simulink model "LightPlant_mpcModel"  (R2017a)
settings: Solver=VariableStepAuto  StartTime=0.0  StopTime=100  RelTol=1e-3
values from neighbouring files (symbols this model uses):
  baud = 250000    [init.m]    (also in steadyState.m; MISOcontrol.m; MISO_demo.m; runSteptest.m)
  com = 'COM4'    [init.m]    (also in steadyState.m; MISOcontrol.m; MISO_demo.m; runSteptest.m)
  fixed_u1 = 0    [init.m]    (also in MISOcontrol.m; MISO_demo.m; SISOcontrol.m)
  fixed_u2 = 0    [init.m]    (also in MISOcontrol.m; MISO_demo.m; SISOcontrol.m)
  fixed_u3 = 0    [init.m]    (also in MISOcontrol.m; MISO_demo.m; SISOcontrol.m)
  fTf = 0.1    [init.m]    (also in steadyState.m; MISOcontrol.m; MISO_demo.m; runSteptest.m)
  fTl = 0.05    [init.m]    (also in steadyState.m; MISOcontrol.m; MISO_demo.m; runSteptest.m)
  fTt = 0.05    [init.m]    (also in steadyState.m; MISOcontrol.m; MISO_demo.m; runSteptest.m)
  step_ys1_1 = +0    (= 0)    [init.m]    (also in LightPlantMPC.m = 1; MIMOcontrol.m = -2)
  step_ys1_2 = -0    (= 0)    [init.m]    (also in LightPlantMPC.m = -1; MIMOcontrol.m)
  step_ys2_1 = 0    [init.m]    (also in LightPlantMPC.m = 5; MIMOcontrol.m = -20)
  step_ys2_2 = 0    [init.m]    (also in LightPlantMPC.m = -5; MIMOcontrol.m = 10)
  stepTime_ys1_1 = 0    [init.m]    (also in LightPlantMPC.m = 30; MIMOcontrol.m = 60)
  stepTime_ys1_2 = 0    [init.m]    (also in LightPlantMPC.m = 70; MIMOcontrol.m)
  stepTime_ys2_1 = 0    [init.m]    (also in LightPlantMPC.m = 20; MIMOcontrol.m = 30)
  stepTime_ys2_2 = 0    [init.m]    (also in LightPlantMPC.m = 50; MIMOcontrol.m = 90)
  Ts = 0.1    [init.m]    (also in steadyState.m; identification.m; MISOcontrol.m; MISO_demo.m)
undefined symbols (not defined in the file or in its folder): A, B, C, D, stst
libraries: mpclib x1, tom_lib x1

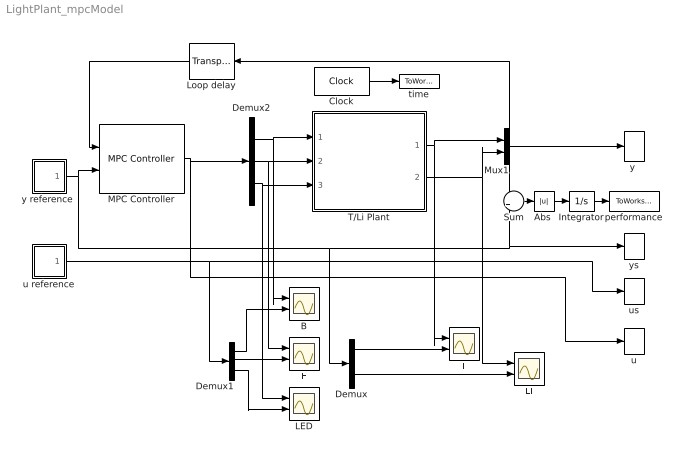
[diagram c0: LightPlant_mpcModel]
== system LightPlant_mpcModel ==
  "Abs " : Abs  ZeroCross=off
  B : Scope  NumInputPorts=2
  Clock : Clock
  Demux : Demux  Outputs=2
  Demux1 : Demux  Outputs=3
  Demux2 : Demux  Outputs=3
  F : Scope  NumInputPorts=2
  Integrator : Integrator  ZeroCross=off
  LED : Scope  NumInputPorts=2
  LI : Scope  NumInputPorts=2
  Loop delay : TransportDelay  DelayTime=0.1
  MPC Controller : mpclib/MPC Controller  SCDEnableBlockLinearizationSpecification=on  mpcobj=MPCobj  is_multiple=0  enable_value=0  return_u0=off  ref_from_ws=off  ref_signal_name=[]  ref_preview=off  md_from_ws=off  md_signal_name=[]  md_preview=off  from_project=off  project_file=MPCtask.mat  md_inport=off  mv_inport=off  cost_outport=off  return_sequence=off  return_qpstatus=off  return_state=off  state_inport=off  lims_inport=off  ywt_inport=off  is_designfromscratch=0  uwt_inport=off  duwt_inport=off  rhoeps_inport=off  uref_inport=off  n_ts=0.1  n_mv=3  n_md=0  n_ud=0  n_mo=2  n_uo=0  BlockDataType=double  SampleTimeInherited=off  switch_inport=off
  Mux1 : Mux  Inputs=2
  Sum : Sum  Inputs=-+
  T : Scope  NumInputPorts=2
  T/Li Plant : Subsystem
  performance : ToWorkspace  VariableName=IAE  SampleTime=Ts
  time : ToWorkspace  VariableName=time  SampleTime=Ts
  u : ToWorkspace  VariableName=u  SampleTime=Ts
  u reference : Subsystem
  us : ToWorkspace  VariableName=us  SampleTime=Ts
  "y " : ToWorkspace  VariableName=y  SampleTime=Ts
  "y reference " : Subsystem
  ys : ToWorkspace  VariableName=ys  SampleTime=Ts
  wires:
  Demux2/2 -> T/Li Plant/2(F), F/1
  Demux2/1 -> B/1, T/Li Plant/1(B)
  "y reference "/1(ys) -> Demux/1, Sum/2, ys/1, MPC Controller/2
  Demux2/3 -> LED/1, T/Li Plant/3(LED)
  T/Li Plant/1(T) -> T/1, Mux1/1
  Loop delay/1 -> MPC Controller/1
  T/Li Plant/2(LI) -> LI/1, Mux1/2
  Mux1/1 -> "y "/1, Sum/1, Loop delay/1
  MPC Controller/1 -> u/1, Demux2/1
  Demux/1 -> T/2
  Demux/2 -> LI/2
  u reference/1(us) -> Demux1/1, us/1
  Demux1/1 -> B/2
  Demux1/2 -> F/2
  Demux1/3 -> LED/2
  Clock/1 -> time/1
  "Abs "/1 -> Integrator/1
  Integrator/1 -> performance/1
  Sum/1 -> "Abs "/1

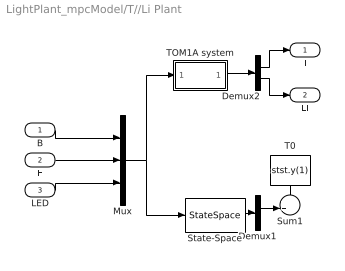
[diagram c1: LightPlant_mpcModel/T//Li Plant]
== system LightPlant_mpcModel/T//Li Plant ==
  B : Inport
  F : Inport  Port=2
  LED : Inport  Port=3
  Demux1 : Demux  Commented=on  Outputs=2
  Demux2 : Demux  Outputs=2
  Mux : Mux  Inputs=3
  State-Space : StateSpace  Commented=on  A=A  B=B  C=C  D=D  X0=0
  Sum1 : Sum  Commented=on  Inputs=++|
  T0 : Constant  Commented=on  Value=stst.y(1)
  TOM1A system : Subsystem
  T : Outport
  LI : Outport  Port=2
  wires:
  B/1 -> Mux/1
  F/1 -> Mux/2
  LED/1 -> Mux/3
  Mux/1 -> TOM1A system/1(u), State-Space/1
  State-Space/1 -> Demux1/1
  T0/1 -> Sum1/1
  Demux1/1 -> Sum1/2
  Sum1/1 -> ?
  TOM1A system/1(y) -> Demux2/1
  Demux2/1 -> T/1
  Demux2/2 -> LI/1

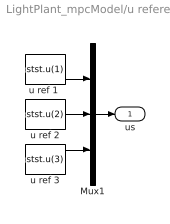
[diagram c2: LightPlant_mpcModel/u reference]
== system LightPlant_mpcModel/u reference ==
  Mux1 : Mux  Inputs=3
  "u ref 1 " : Constant  Value=stst.u(1)  SampleTime=Ts
  u ref 2 : Constant  Value=stst.u(2)  SampleTime=Ts
  u ref 3 : Constant  Value=stst.u(3)  SampleTime=Ts
  us : Outport
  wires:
  u ref 3/1 -> Mux1/3
  "u ref 1 "/1 -> Mux1/1
  u ref 2/1 -> Mux1/2
  Mux1/1 -> us/1

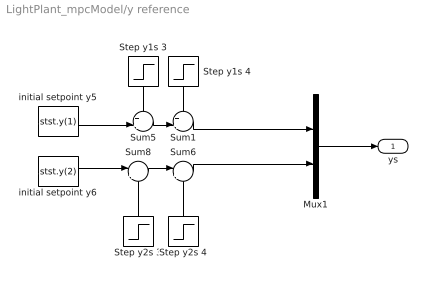
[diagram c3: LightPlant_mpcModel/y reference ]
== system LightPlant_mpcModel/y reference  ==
  Mux1 : Mux  Inputs=2
  Step y1s 3 : Step  Time=stepTime_ys1_1  After=step_ys1_1  SampleTime=Ts  ZeroCross=off
  Step y1s 4 : Step  Time=stepTime_ys1_2  After=step_ys1_2  SampleTime=Ts  ZeroCross=off
  Step y2s 3 : Step  Time=stepTime_ys2_1  After=step_ys2_1  SampleTime=Ts  ZeroCross=off
  Step y2s 4 : Step  Time=stepTime_ys2_2  After=step_ys2_2  SampleTime=Ts  ZeroCross=off
  Sum1 : Sum  Inputs=++|
  Sum5 : Sum  Inputs=++|
  Sum6 : Sum  Inputs=|++
  Sum8 : Sum  Inputs=|++
  initial setpoint y5 : Constant  Value=stst.y(1)  SampleTime=Ts
  initial setpoint y6 : Constant  Value=stst.y(2)  SampleTime=Ts
  ys : Outport
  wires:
  Step y2s 4/1 -> Sum6/2
  Step y1s 3/1 -> Sum5/1
  initial setpoint y6/1 -> Sum8/1
  Sum8/1 -> Sum6/1
  Mux1/1 -> ys/1
  initial setpoint y5/1 -> Sum5/2
  Step y2s 3/1 -> Sum8/2
  Step y1s 4/1 -> Sum1/1
  Sum5/1 -> Sum1/2
  Sum6/1 -> Mux1/2
  Sum1/1 -> Mux1/1

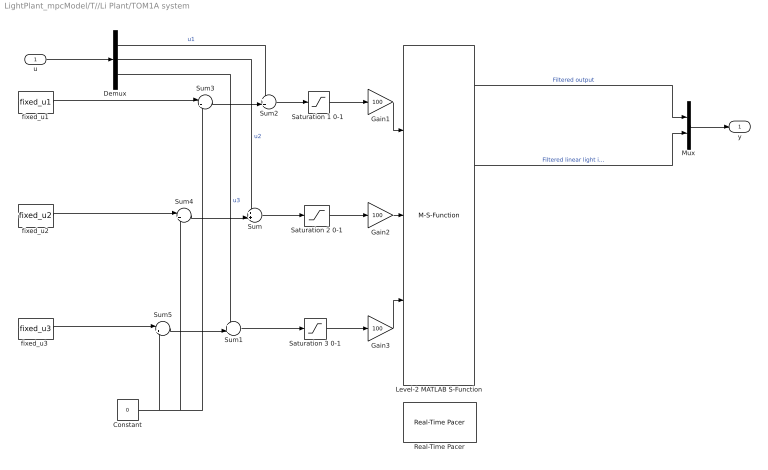
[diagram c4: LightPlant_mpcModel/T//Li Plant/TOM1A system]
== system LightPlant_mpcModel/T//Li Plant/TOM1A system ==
  u : Inport
  Constant : Constant  Value=0
  Demux : Demux  Outputs=3
  Gain1 : Gain  Gain=100
  Gain2 : Gain  Gain=100
  Gain3 : Gain  Gain=100
  Level-2 MATLAB S-Function : M-S-Function  FunctionName=tom1ar8  Parameters=Ts,com,baud,fTt,fTl,fTf
  Mux : Mux  Inputs=2
  Real-Time Pacer : tom_lib/Real-Time Pacer  simTimePerRealTime=1
  "Saturation 1 0-1 " : Saturate  UpperLimit=1  LowerLimit=0  ZeroCross=off
  Saturation 2 0-1 : Saturate  UpperLimit=1  LowerLimit=0  ZeroCross=off
  Saturation 3 0-1 : Saturate  UpperLimit=1  LowerLimit=0  ZeroCross=off
  Sum : Sum  Inputs=++|
  Sum1 : Sum  Inputs=++|
  Sum2 : Sum  Inputs=++|
  Sum3 : Sum  Inputs=|++
  Sum4 : Sum  Inputs=|++
  Sum5 : Sum  Inputs=|++
  fixed_u1 : Constant  Value=fixed_u1  SampleTime=Ts
  fixed_u2 : Constant  Value=fixed_u2  SampleTime=Ts
  "fixed_u3 " : Constant  Value=fixed_u3  SampleTime=Ts
  y : Outport
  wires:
  Level-2 MATLAB S-Function/14 -> ?  "Fan filtered  rpm"
  Level-2 MATLAB S-Function/3 -> ?  "Derivative of internal temperature"
  Level-2 MATLAB S-Function/4 -> ?  "Filtered external temperature"
  Level-2 MATLAB S-Function/13 -> ?  "Fan voltage"
  Level-2 MATLAB S-Function/11 -> ?  "Bulb voltage"
  Level-2 MATLAB S-Function/8 -> ?  "Filtered logaritmic light intensity"
  Level-2 MATLAB S-Function/1 -> ?  "Board temperature"
  Level-2 MATLAB S-Function/5 -> ?  "Derivate of external temperature"
  Level-2 MATLAB S-Function/12 -> ?  "Fan current"
  Level-2 MATLAB S-Function/9 -> ?  "Derivate of logaritmic light intensity"
  Level-2 MATLAB S-Function/16 -> ?  "Count of fan rpm"
  Level-2 MATLAB S-Function/15 -> ?  "Derivate of fan rpm"
  Level-2 MATLAB S-Function/10 -> ?  "Bulb current"
  Level-2 MATLAB S-Function/6 -> Mux/2  "Filtered linear light intensity"
  Level-2 MATLAB S-Function/7 -> ?  "Derivate of linear light intensity"
  Demux/1 -> Sum2/1  "u1"
  Demux/2 -> Sum/1  "u2"
  Demux/3 -> Sum1/1  "u3"
  u/1 -> Demux/1
  Level-2 MATLAB S-Function/2 -> Mux/1  "Filtered output"
  Mux/1 -> y/1
  fixed_u1/1 -> Sum3/1
  Sum3/1 -> Sum2/2
  Constant/1 -> Sum5/2, Sum4/2, Sum3/2
  fixed_u2/1 -> Sum4/1
  "fixed_u3 "/1 -> Sum5/1
  Sum5/1 -> Sum1/2
  Sum4/1 -> Sum/2
  Gain1/1 -> Level-2 MATLAB S-Function/1
  Gain2/1 -> Level-2 MATLAB S-Function/2
  Gain3/1 -> Level-2 MATLAB S-Function/3
  Saturation 2 0-1/1 -> Gain2/1
  Sum/1 -> Saturation 2 0-1/1
  Sum2/1 -> "Saturation 1 0-1 "/1
  Saturation 3 0-1/1 -> Gain3/1
  Sum1/1 -> Saturation 3 0-1/1
  "Saturation 1 0-1 "/1 -> Gain1/1
